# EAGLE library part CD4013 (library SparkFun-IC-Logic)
Dual D-type Flip-Flop Datasheet SparkFun Products SparkFun SparkPunk Sound Kit (KIT-11177) SparkFun SparkPunk Sequencer Kit (KIT-12707)
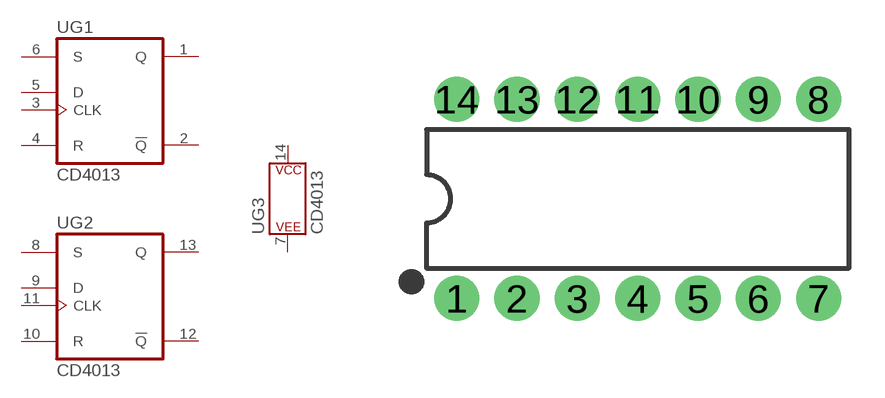
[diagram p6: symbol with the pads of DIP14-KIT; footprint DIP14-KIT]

Designator prefix U; gates G1=CD4013 G2=CD4013 G3=POWER_CONSORT

## CD4013 (PROD_ID: IC-11896; VALUE: CD4013B)  [DIP14-KIT]
1  G1:Q  out
2  G1:!Q  out
3  G1:CLK  in
4  G1:R  in
5  G1:D  in
6  G1:S  in
7  G3:P$V-
8  G2:S  in
9  G2:D  in
10  G2:R  in
11  G2:CLK  in
12  G2:!Q  out
13  G2:Q  out
14  G3:P$V+

## Footprint DIP14-KIT (pad centres in mm)
drill 0.864 pad 1.905: 1 -8.89,-4.191; 2 -6.35,-4.191; 3 -3.81,-4.191; 4 -1.27,-4.191; 5 1.27,-4.191; 6 3.81,-4.191; 7 6.35,-4.191; 8 6.35,4.191; 9 3.81,4.191; 10 1.27,4.191; 11 -1.27,4.191; 12 -3.81,4.191; 13 -6.35,4.191; 14 -8.89,4.191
